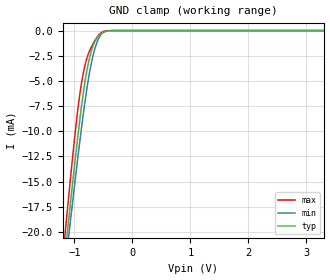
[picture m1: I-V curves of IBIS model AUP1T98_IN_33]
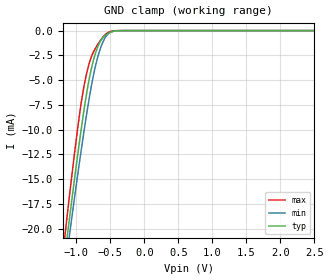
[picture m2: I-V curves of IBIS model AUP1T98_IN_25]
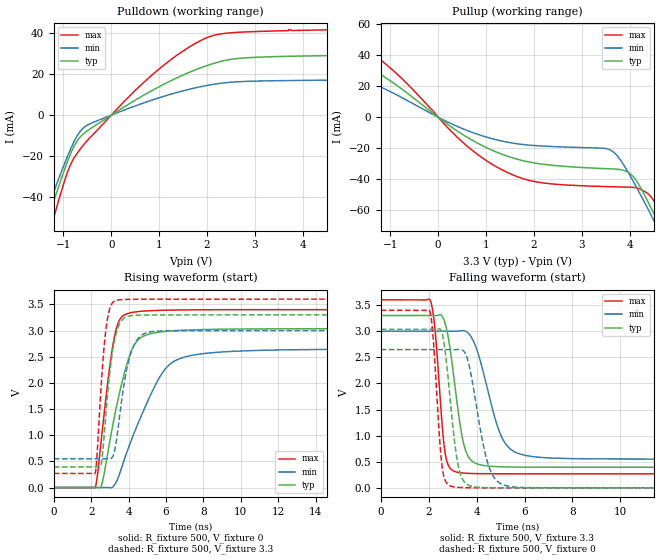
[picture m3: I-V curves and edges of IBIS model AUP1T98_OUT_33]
| TEXAS INSTRUMENTS INCORPORATED
| Standard Linear and Logic Group
| IBIS Model of SN74AUP1T98
| SINGLE-SUPPLY VOLTAGE TRANSLATOR
| This file contains package information for the following:
|  SOT 6-pin (DBV) package as [Component] AUP1T98_DBV
|  SOT 6-pin (DCK) package as [Component] AUP1T98_DCK
|  DSBGA 6-pin (YZP) package as [Component] AUP1T98_YZP
| This device can be powered at the following Vccs:
|  3.3 volt Vcc
|  2.5 volt Vcc
| This file provides unique models under the [Model Selector] for each Vcc.
| For operation at a specific Vcc, select the appropriate model after each
| [Model Selector] keyword.
[IBIS Ver]   3.2
[Comment char]  |_char
[File Name]   sn74aup1t98.ibs
[File Rev]   1.2 | x_die
[Date]   December 7, 2005
[Source]   Data created from TI-SPICE simulations at TI-SLL.
[Notes]   The following is an IBIS list for the AUP1T98.
   Please contact sllibis@ti.com with questions and
   comments concerning SLL IBIS models.
   - FILE REV HISTORY
   - 1.1 Release IBIS file on 10/01/04
   - 1.2 YZP package added on 12/07/05
   - Non-monotonic data in pullup due to special output circuit.
   - Power clamp data deleted as there is no power-clamp diode.
[Disclaimer] Property of Texas Instruments Incorporated.  Unauthorized
   reproduction and/or distribution is strictly prohibited.
   This product is protected under copyright law.
   Created  2004, (C) Copyright  2004, Texas Instruments
   Incorporated, All Rights Reserved
   UNLESS THERE IS A SIGNED, WRITTEN AGREEMENT TO THE
   CONTRARY, TEXAS INSTRUMENTS (TI) IS PROVIDING THE IBIS
   MODELS  AND WITHOUT ANY WARRANTY, EXPRESSED OR
   IMPLIED.  TI assumes no liability for:
   1) the accuracy of the IBIS models provided to your
   company;
   2) the proper functioning of these IBIS Models in your
   design or for any resulting applications; or
   3) infringement of patents, copyrights or intellectual
   property rights resulting from your use of these IBIS
   models.
   TI provides IBIS Models as a service to our customers.
   You and your company shall not distribute, sell or give
   these models to anyone else without prior written
   permission from TI.
   TI reserves the right to make changes to our products or
   to discontinue any semiconductor product or service
   without notice, and advises our customers to obtain the
   latest version of relevant information to verify, before
   placing orders, that the information being relied on is
   current.
   Please be aware that your receipt and use of the IBIS
   information provided shall serve as acceptance of these
   terms and conditions.  If you do not accept these terms,
   you should return or destroy the IBIS models and any
   other accompanying information immediately.
| Component AUP1T98_DBV 6-pin SOT
[Component]   AUP1T98_DBV
[Manufacturer]   Texas Instruments, Inc.
[Package]
|   typ   min   max
R_pkg   2.500e-02   1.900e-02   3.700e-02
L_pkg   1.524e-09   1.260e-09   1.751e-09
C_pkg   2.450e-13   1.980e-13   2.640e-13
[Pin]   signal_name   model_name   R_pin   L_pin   C_pin
1   B   AUP1T98_IN   2.100e-02   1.405e-09   2.460e-13
2   GND   GND   3.700e-02   1.751e-09   2.630e-13
3   A   AUP1T98_IN   2.600e-02   1.493e-09   2.470e-13
4   y   AUP1T98_OUT   1.900e-02   1.620e-09   2.640e-13
5   VCC   POWER   2.400e-02   1.260e-09   1.980e-13
6   C   AUP1T98_IN   2.100e-02   1.617e-09   2.500e-13
| Component AUP1T98_DCK 6-pin SOT
[Component]   AUP1T98_DCK
[Manufacturer]   Texas Instruments, Inc.
[Package]
|   typ   min   max
R_pkg   1.400e-02   1.100e-02   2.100e-02
L_pkg   9.480e-10   7.840e-10   1.103e-09
C_pkg   1.910e-13   1.670e-13   2.050e-13
[Pin]   signal_name   model_name   R_pin   L_pin   C_pin
1   B   AUP1T98_IN   1.300e-02   9.840e-10   1.960e-13
2   GND   GND   2.100e-02   1.103e-09   2.050e-13
3   A   AUP1T98_IN   1.100e-02   9.980e-10   1.970e-13
4   Y   AUP1T98_OUT   1.300e-02   9.040e-10   1.900e-13
5   VCC   POWER   1.500e-02   7.840e-10   1.670e-13
6   C   AUP1T98_IN   1.200e-02   9.160e-10   1.950e-13
| Component AUP1T98_YZP 6-pin DSBGA
[Component]   AUP1T98_YZP
[Manufacturer]   Texas Instruments, Inc.
[Package]
|   typ   min   max
R_pkg   1.000e-03   1.000e-03   2.100e-02
L_pkg   2.450e-11   2.400e-11   1.103e-09
C_pkg   5.600e-14   0.000e+00   2.050e-13
[Pin]   signal_name   model_name   R_pin   L_pin   C_pin
1   B   AUP1T98_IN   1.000e-03   2.500e-11   6.400e-14
2   GND   GND   1.000e-03   2.400e-11   6.700e-14
3   A   AUP1T98_IN   1.000e-03   2.500e-11   6.400e-14
4   Y   AUP1T98_OUT   1.000e-03   2.500e-11   6.400e-14
5   VCC   POWER   1.000e-03   2.400e-11   6.700e-14
6   C   AUP1T98_IN   1.000e-03   2.500e-11   6.400e-14
| Model AUP1T98_IN
[Model Selector]   AUP1T98_IN
AUP1T98_IN_33   3.3 volt Vcc
AUP1T98_IN_25   2.5 volt Vcc
| Model AUP1T98_OUT
[Model Selector]   AUP1T98_OUT
AUP1T98_OUT_33   3.3 volt Vcc
AUP1T98_OUT_25   2.5 volt Vcc
| Models and submodels in the file (4): AUP1T98_IN_33 (Input), AUP1T98_IN_25 (Input), AUP1T98_OUT_33 (Output), AUP1T98_OUT_25 (Output)
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[Model]   AUP1T98_IN_33
Model_type  Input
Vinl=0.9
Vinh=2.1
| variable   typ   min   max
C_comp   1.42pF   1.16pF   1.79pF
[Temperature Range]   40   100   -40
| Ambient temperature   25   85   -40
[Voltage range]   3.3   3   3.6
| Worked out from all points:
|   GND clamp passes 1 mA (typ) near -0.64 V on its own axis
[GND Clamp]
| AUP1T98_IN_33
|   Voltage   I(typ)   I(min)   I(max)
-3.6V     -171.6mA   -163.5mA   -181.1mA
-1.16V    -22.22mA   -23.69mA   -20.18mA
-1.11V    -19.45mA   -21.09mA   -17.19mA
-1.085V   -18.08mA   -19.81mA   -15.71mA
-940mV    -10.5mA    -12.6mA    -7.822mA
-890mV    -8.117mA   -10.26mA   -5.698mA
-835mV    -5.768mA   -7.825mA   -3.925mA
-755mV    -3.153mA   -4.717mA   -2.255mA
-675mV    -1.463mA   -2.419mA   -1.277mA
-595mV    -617.7uA   -945.8uA   -546.7uA
-515mV    -215.4uA   -248.8uA   -134.4uA
3.3V      132.2pA    540.4pA    36.28pA
[Model]   AUP1T98_IN_25
Model_type  Input
Vinl=0.7
Vinh=1.6
| variable   typ   min   max
C_comp   1.46pF   1.21pF   1.78pF
[Temperature Range]   40   100   -40
| Ambient temperature   25   85   -40
[Voltage range]   2.5   2.3   2.7
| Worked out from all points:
|   GND clamp passes 1 mA (typ) near -0.64 V on its own axis
[GND Clamp]
| AUP1T98_IN_25
|   Voltage   I(typ)   I(min)   I(max)
-3.6V     -171.6mA   -163.5mA   -181.1mA
-1.165V   -22.5mA    -23.95mA   -20.48mA
-1.115V   -19.72mA   -21.35mA   -17.49mA
-1.09V    -18.36mA   -20.06mA   -16.01mA
-945mV    -10.75mA   -12.84mA   -8.061mA
-890mV    -8.117mA   -10.26mA   -5.698mA
-835mV    -5.768mA   -7.825mA   -3.925mA
-760mV    -3.287mA   -4.89mA    -2.329mA
-675mV    -1.463mA   -2.419mA   -1.277mA
-595mV    -617.7uA   -945.8uA   -546.7uA
-520mV    -233.1uA   -272.6uA   -149.9uA
2.5V      104.3pA    491.9pA    26.71pA
[Model]   AUP1T98_OUT_33
Model_type  Output
Vref =   0
Rref =   1E6
Cref =   30p
Vmeas =   1.65
| variable   typ   min   max
C_comp   2.73pF   1.81pF   4.12pF
| C_pullup   3.12pF   1.81pF   4.12pF
| C_pulldown   2.33pF   2.13pF   2.90pF
[Temperature Range]   40   100   -40
| Ambient temperature   25   85   -40
[Voltage range]   3.3   3   3.6
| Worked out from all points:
|   slope of the pulldown table from 0 to 0.495 V, typ, clamps not added: 68.4 ohm
|   slope of the pullup table from 0 to 0.495 V, typ, clamps not added: 45.8 ohm
|   rising waveform, R_fixture 500, V_fixture 0: 20-80 % time 1.11ns typ, 1.91ns min, 689ps max; typ from 0 V to 3.04 V
|   falling waveform, R_fixture 500, V_fixture 3.3: 20-80 % time 524ps typ, 876ps min, 331ps max; typ from 3.3 V to 0.394 V
|   rising waveform, R_fixture 500, V_fixture 3.3: 20-80 % time 506ps typ, 667ps min, 393ps max; typ from 0.394 V to 3.3 V
|   falling waveform, R_fixture 500, V_fixture 0: 20-80 % time 427ps typ, 642ps min, 287ps max; typ from 3.04 V to 0 V
[Pulldown]
| AUP1T98_OUT_33
|   Voltage   I(typ)   I(min)   I(max)
-3.6V     -218.7mA   -196.3mA   -248.6mA
-1.515V   -64.37mA   -57.31mA   -75.82mA
-1.39V    -55.35mA   -49.29mA   -65.41mA
-1.275V   -47.14mA   -42mA      -55.89mA
-870mV    -19.93mA   -17.62mA   -25.18mA
-720mV    -12.85mA   -10.38mA   -18.82mA
-545mV    -8.444mA   -5.509mA   -13.51mA
940mV     13.13mA    8.018mA    21.36mA
1.5V      19.56mA    11.86mA    31.27mA
2.045V    24.53mA    14.67mA    38.2mA
3.1V      28.27mA    16.63mA    40.81mA
7.2V      29.73mA    17.36mA    42.67mA
[Pullup]
| AUP1T98_OUT_33
|   Voltage   I(typ)   I(min)   I(max)
-3.6V     42.88mA    27.27mA    57.92mA
-2.465V   31.53mA    19.52mA    45.85mA
-1.53V    32.87mA    22.09mA    44.95mA
-755mV    18.1mA     12.64mA    24.89mA
555mV     -11.98mA   -7.942mA   -17.3mA
1.65V     -27.07mA   -17.13mA   -38.31mA
3.61V     -33.32mA   -21.39mA   -44.82mA
4.08V     -38.63mA   -41.77mA   -45.28mA
4.375V    -54.25mA   -58.9mA    -49.24mA
4.565V    -66.24mA   -70.37mA   -57.33mA
4.775V    -80.02mA   -83.29mA   -71.37mA
7.2V      -250.7mA   -240.9mA   -257mA
[Ramp]
| AUP1T98_OUT_33
| variable   typ   min   max
dV/dt_r   1.82/1.11E-09   1.59/1.91E-09   2.04/6.91E-10
dV/dt_f   1.75/5.30E-10   1.48/8.84E-10   2.01/3.34E-10
R_load = 500
[Rising Waveform]
| AUP1T98_OUT_33
R_fixture =   500
C_fixture =   0
L_fixture =   0
V_fixture =   0
V_fixture_min = 0
V_fixture_max = 0
|   Time   V(typ)   V(min)   V(max)
0s        24.73nV    82.54nV    2.123nV
2.215ns   -65.09uV   162nV      4.401mV
2.585ns   89.78mV    -115uV     1.065V
3.215ns   1.308V     33.98mV    2.833V
3.5ns     1.79V      245.6mV    3.193V
3.96ns    2.421V     729.8mV    3.326V
4.56ns    2.838V     1.272V     3.364V
5.79ns    2.976V     2.183V     3.387V
7.3ns     3.012V     2.52V      3.395V
29.99ns   3.035V     2.647V     3.399V
[Falling Waveform]
| AUP1T98_OUT_33
R_fixture =   500
C_fixture =   0
L_fixture =   0
V_fixture =   3.3
V_fixture_min = 3
V_fixture_max = 3.6
|   Time   V(typ)   V(min)   V(max)
0s        3.3V       3V         3.6V
2.075ns   3.3V       3V         3.582V
2.265ns   3.299V     3V         3.035V
2.68ns    3.16V      3V         693.5mV
3.16ns    1.719V     2.999V     302.9mV
3.445ns   875.7mV    3.012V     283.6mV
3.76ns    533.9mV    2.901V     275.7mV
5.03ns    403.6mV    989.5mV    269.8mV
6.055ns   396.4mV    619.7mV    269.4mV
29.99ns   394.1mV    550mV      269.3mV
[Rising Waveform]
| AUP1T98_OUT_33
R_fixture =   500
C_fixture =   0
L_fixture =   0
V_fixture =   3.3
V_fixture_min = 3
V_fixture_max = 3.6
|   Time   V(typ)   V(min)   V(max)
0s        394.1mV    550mV      269.3mV
2.215ns   394mV      550mV      280.5mV
2.535ns   455.1mV    550mV      1.958V
2.77ns    1.34V      551.2mV    2.973V
3.04ns    2.341V     551.7mV    3.466V
3.31ns    2.915V     819.8mV    3.575V
3.75ns    3.236V     1.965V     3.593V
4.07ns    3.28V      2.513V     3.596V
5.065ns   3.296V     2.968V     3.599V
29.99ns   3.3V       3V         3.6V
[Falling Waveform]
| AUP1T98_OUT_33
R_fixture =   500
C_fixture =   0
L_fixture =   0
V_fixture =   0
V_fixture_min = 0
V_fixture_max = 0
|   Time   V(typ)   V(min)   V(max)
0s        3.035V     2.647V     3.399V
2.05ns    3.035V     2.647V     3.379V
2.195ns   3.035V     2.647V     2.833V
2.555ns   2.975V     2.647V     431.7mV
2.985ns   1.288V     2.647V     23.54mV
3.225ns   447.4mV    2.649V     9.182mV
3.5ns     107.2mV    2.597V     3.703mV
4.485ns   3.329mV    446.5mV    218.2uV
5.295ns   514.9uV    33.55mV    36.26uV
29.99ns   -2.167nV   142.2nV    -10.93nV
